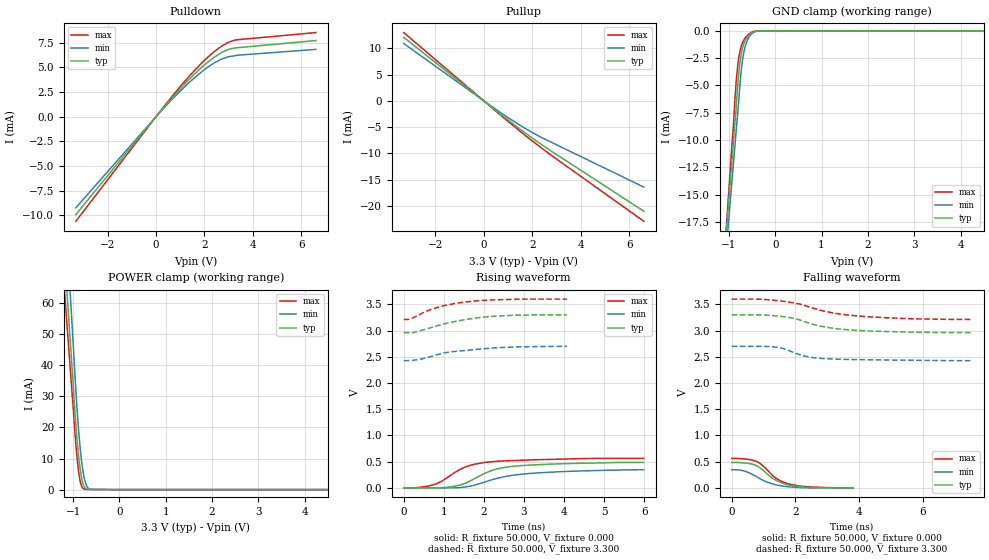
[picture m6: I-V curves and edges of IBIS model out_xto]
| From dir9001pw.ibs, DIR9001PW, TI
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[Model]   out_xto
Model_type Output
Vref=0.000E+00
Rref=1.000E+06
Cref=2.000E-11
Vmeas=1.650E+00
C_comp   660.0fF   660.0fF   660.0fF
[Voltage Range]   3.300E+00   2.700E+00   3.600E+00
[POWER Clamp Reference]   3.300E+00   2.700E+00   3.600E+00
[GND Clamp Reference]   0.000E+00   0.000E+00   0.000E+00
[Pullup Reference]   3.300E+00   2.700E+00   3.600E+00
[Pulldown Reference]   0.000E+00   0.000E+00   0.000E+00
[Temperature Range]   25   85   -40
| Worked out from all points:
|   slope of the pulldown table from 0 to 0.495 V, typ, clamps not added: 344 ohm
|   slope of the pullup table from 0 to 0.495 V, typ, clamps not added: 270 ohm
|   GND clamp passes 1 mA (typ) near -0.66 V on its own axis
|   POWER clamp passes 1 mA (typ) near -0.76 V on its own axis
|   rising waveform, R_fixture 50.000, V_fixture 0.000: 20-80 % time 941ps typ, 1.35ns min, 851ps max; typ from 0 V to 0.484 V
|   falling waveform, R_fixture 50.000, V_fixture 0.000: 20-80 % time 687ps typ, 735ps min, 692ps max; typ from 0.484 V to 0 V
|   rising waveform, R_fixture 50.000, V_fixture 3.300: 20-80 % time 1.18ns typ, 1.29ns min, 963ps max; typ from 2.96 V to 3.3 V
|   falling waveform, R_fixture 50.000, V_fixture 3.300: 20-80 % time 1.45ns typ, 934ps min, 1.75ns max; typ from 3.3 V to 2.96 V
[GND Clamp]
-3.31V    -139.8mA   -133.5mA   -158.2mA
-930mV    -11.62mA   -13.54mA   -10.14mA
-890mV    -9.462mA   -11.52mA   -7.776mA
-850mV    -7.477mA   -9.516mA   -5.016mA
-830mV    -6.153mA   -8.484mA   -3.984mA
-770mV    -3.176mA   -5.346mA   -2.037mA
-730mV    -2.019mA   -3.487mA   -1.359mA
-670mV    -1.079mA   -1.794mA   -793.1uA
-590mV    -487.7uA   -748uA     -378.4uA
-490mV    -134.6uA   -209.1uA   -90.49uA
-330mV    0A         0A         0A
6.6V      0A         0A         0A
[Power Clamp]
-3.3V     544mA      634.8mA    486mA
-1.02V    38.68mA    52.52mA    30.72mA
-940mV    20.75mA    31.93mA    14.53mA
-900mV    13.4mA     22.91mA    8.143mA
-880mV    10.46mA    18.97mA    5.669mA
-860mV    7.971mA    15.41mA    3.697mA
-820mV    4.004mA    9.522mA    1.254mA
-760mV    902.1uA    3.772mA    173.5uA
-720mV    284.3uA    1.644mA    59.74uA
-680mV    112.3uA    582.1uA    34.83uA
-560mV    44.72uA    50.39uA    25.95uA
6.6V      0A         0A         0A
[Pullup]
-3.3V     12.09mA    10.91mA    13mA
220mV     -819.4uA   -733.5uA   -880.7uA
1.56V     -5.615mA   -4.848mA   -6.036mA
2.4V      -8.39mA    -7.035mA   -9.067mA
6.6V      -21.04mA   -16.44mA   -22.96mA
[Pulldown]
-3.31V    -9.911mA   -9.226mA   -10.59mA
0V        0A         0A         0A
590mV     1.711mA    1.573mA    1.841mA
1.49V     4.088mA    3.733mA    4.424mA
1.91V     5.06mA     4.601mA    5.497mA
2.39V     6.009mA    5.43mA     6.568mA
2.69V     6.479mA    5.822mA    7.117mA
2.95V     6.78mA     6.054mA    7.488mA
3.25V     6.972mA    6.189mA    7.762mA
6.61V     7.731mA    6.835mA    8.539mA
[Rising Waveform]
R_fixture = 50.000
V_fixture = 0.000
V_fixture_min = 0.000
V_fixture_max = 0.000
|  time   V(typ)   V(min)   V(max)
0s        0V         -150.4uV   0V
430ps     0V         -150.4uV   11.75mV
770ps     313.8uV    -150.4uV   66.26mV
940ps     2.084mV    -150.4uV   124.1mV
1.28ns    32.73mV    750uV      295.4mV
1.62ns    116.9mV    27.23mV    419.3mV
2.09ns    299.6mV    127.8mV    490.6mV
2.49ns    385.4mV    209.2mV    513mV
3.13ns    432.9mV    273.3mV    531.2mV
5.99ns    484mV      346mV      561.5mV
[Falling Waveform]
R_fixture = 50.000
V_fixture = 0.000
V_fixture_min = 0.000
V_fixture_max = 0.000
|  time   V(typ)   V(min)   V(max)
0s        484mV      346mV      561.5mV
390ps     475.8mV    322.4mV    552.3mV
790ps     419.9mV    211.2mV    501.9mV
910ps     371.5mV    169mV      457.5mV
1.07ns    289.4mV    120.1mV    369.4mV
1.4ns     141mV      57.28mV    180.5mV
1.57ns    94.51mV    37.6mV     124.5mV
1.85ns    47.04mV    17.35mV    66.67mV
2.47ns    7.351mV    -149.7uV   17.75mV
3.81ns    0V         -150.4uV   0V
[Rising Waveform]
R_fixture = 50.000
V_fixture = 3.300
V_fixture_min = 2.700
V_fixture_max = 3.600
|  time   V(typ)   V(min)   V(max)
0s        2.961V     2.426V     3.213V
170ps     2.961V     2.43V      3.224V
390ps     2.993V     2.449V     3.304V
540ps     3.026V     2.475V     3.361V
800ps     3.084V     2.532V     3.433V
1.13ns    3.148V     2.59V      3.495V
1.57ns    3.214V     2.622V     3.549V
2.44ns    3.282V     2.677V     3.591V
3.25ns    3.3V       2.693V     3.6V
4.07ns    3.3V       2.7V       3.6V
[Falling Waveform]
R_fixture = 50.000
V_fixture = 3.300
V_fixture_min = 2.700
V_fixture_max = 3.600
|  time   V(typ)   V(min)   V(max)
0s        3.3V       2.7V       3.6V
850ps     3.299V     2.7V       3.599V
1.42ns    3.279V     2.682V     3.573V
1.92ns    3.238V     2.588V     3.532V
2.32ns    3.164V     2.51V      3.474V
2.96ns    3.066V     2.463V     3.363V
3.57ns    3.02V      2.45V      3.302V
4.38ns    2.991V     2.442V     3.26V
5.61ns    2.971V     2.435V     3.226V
7.54ns    2.961V     2.426V     3.213V
[Ramp]
dV/dt_r   2.9056E-01/9.4012E-10   2.0757E-01/1.3454E-09   3.3688E-01/8.4930E-10
dV/dt_f   2.0366E-01/1.4437E-09   1.6442E-01/9.2641E-10   2.3215E-01/1.7534E-09
R_load = 50
